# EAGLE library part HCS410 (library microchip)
ENCODER code hopping encoder and transponder
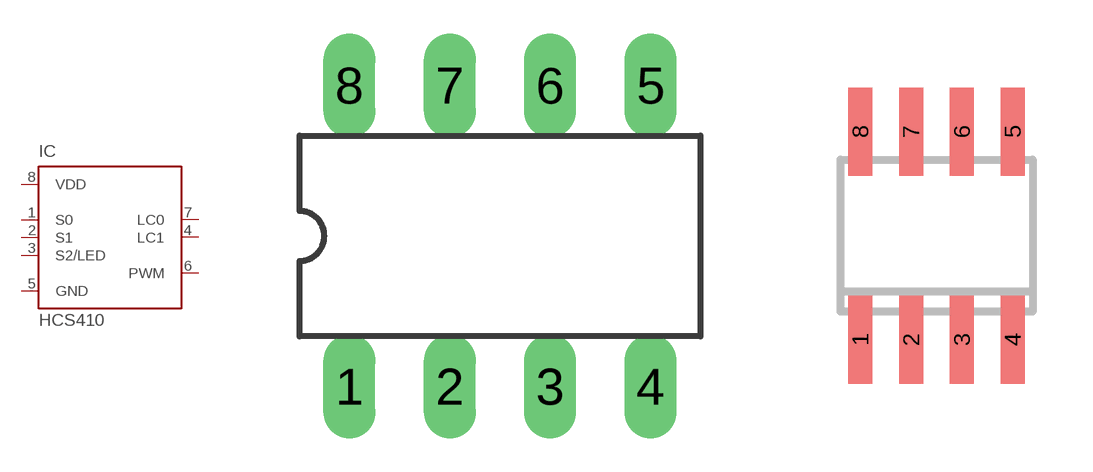
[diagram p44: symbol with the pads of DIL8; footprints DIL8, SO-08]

Designator prefix IC

## HCS410P (MF: MICROCHIP; MPN: HCS410-I/P; OC_FARNELL: unknown; OC_NEWARK: 96K3679)  [DIL8]
1  S0  in
2  S1  in
3  S2/LED
4  LC1
5  GND  pwr
6  PWM
7  LC0
8  VDD  pwr

## HCS410SO (OC_FARNELL: unknown; OC_NEWARK: unknown)  [SO-08]
Pads as for DIL8

## HCS410TS (MF: MICROCHIP; MPN: HCS410-I/ST; OC_FARNELL: unknown; OC_NEWARK: 33C0783)  [TSSOP8]
1  S2/LED
2  LC1
3  GND  pwr
4  PWM
5  LC0
6  VDD  pwr
7  S0  in
8  S1  in

## Footprint DIL8 (pad centres in mm)
Dual In Line package type P
drill 0.813 long: 1 -3.81,-3.81; 2 -1.27,-3.81; 3 1.27,-3.81; 4 3.81,-3.81; 5 3.81,3.81; 6 1.27,3.81; 7 -1.27,3.81; 8 -3.81,3.81

## Footprint SO-08 (pad centres in mm)
Small Outline Narrow Plastic Gull Wing 150-mil body, package type SN
smd 0.6 x 2.2: 1 -1.905,-2.6; 2 -0.635,-2.6; 3 0.635,-2.6; 4 1.905,-2.6; 5 1.905,2.6; 6 0.635,2.6; 7 -0.635,2.6; 8 -1.905,2.6

## Footprint TSSOP8 (pad centres in mm)
Thin Shrink Small Outline Package package type ST
smd 0.35 x 1.2: 1 -0.975,-2.925; 2 -0.325,-2.925; 3 0.325,-2.925; 4 0.975,-2.925; 5 0.975,2.925; 6 0.325,2.925; 7 -0.325,2.925; 8 -0.975,2.925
